DATA_BLOCK "Telegramindeling"
TITLE =
VERSION : 0.1


  STRUCT
   Telegram3 : STRUCT
    hoogwater : BOOL ;
    laagwater : BOOL ;
    water_op_vloer : BOOL ;
    lenspomp_1_stor : BOOL ;
    gereserveerd : BOOL ;
    niveaumeter_1_stor : BOOL ;
    analoge_ingang_1_stor : BOOL ;
    niveaumeter_2_stor : BOOL ;
    analoge_ingang_2_stor : BOOL ;
    verzamelstor_pompen : BOOL ;
    regenpompen_in : BOOL ;
    regenpompen_uit : BOOL ;
    inbraakalarm : BOOL ;
    debietmeter_stor : BOOL ;
    droogloop_elektrode : BOOL ;
    drukknop_herstel_stor : BOOL ;
   END_STRUCT ;
   Telegram4 : STRUCT
    pomp_1_thermistor_stor : BOOL ;
    pomp_1_terugmelding : BOOL ;
    pomp_1_looptijd_te_lang : BOOL ;
    pomp_1_thermische_stor : BOOL ;
    pomp_2_thermistor_stor : BOOL ;
    pomp_2_terugmelding : BOOL ;
    pomp_2_looptijd_te_lang : BOOL ;
    pomp_2_thermische_stor : BOOL ;
    pomp_3_thermistor_stor : BOOL ;
    pomp_3_terugmelding : BOOL ;
    pomp_3_looptijd_te_lang : BOOL ;
    pomp_3_thermische_stor : BOOL ;
    overstorthoogte_bereikt : BOOL ;
    gereserveerd1 : BOOL ;
    vlotterbal_kelder1_hoog : BOOL ;
    gereserveerd2 : BOOL ;
   END_STRUCT ;
   Telegram5 : STRUCT
    pomp_4_thermistor_stor : BOOL ;
    pomp_4_terugmelding : BOOL ;
    pomp_4_looptijd_te_lang : BOOL ;
    pomp_4_thermische_stor : BOOL ;
    pomp_5_thermistor_stor : BOOL ;
    pomp_5_terugmelding : BOOL ;
    pomp_5_looptijd_te_lang : BOOL ;
    pomp_5_thermische_stor : BOOL ;
    pomp_6_thermistor_stor : BOOL ;
    pomp_6_terugmelding : BOOL ;
    pomp_6_looptijd_te_lang : BOOL ;
    pomp_6_thermische_stor : BOOL ;
    procesafsluiter_stor : BOOL ;
    netwachter_stor : BOOL ;
    stuurstroom_stor : BOOL ;
    gereserveerd1 : BOOL ;
   END_STRUCT ;
   Telegram6 : STRUCT
    gereserveerd1 : BOOL ;
    gereserveerd2 : BOOL ;
    gereserveerd3 : BOOL ;
    gereserveerd4 : BOOL ;
    gereserveerd5 : BOOL ;
    gereserveerd6 : BOOL ;
    gereserveerd7 : BOOL ;
    gereserveerd8 : BOOL ;
    gereserveerd9 : BOOL ;
    gereserveerd10 : BOOL ;
    gereserveerd11 : BOOL ;
    gereserveerd12 : BOOL ;
    gereserveerd13 : BOOL ;
    gereserveerd14 : BOOL ;
    gereserveerd15 : BOOL ;
    gereserveerd16 : BOOL ;
   END_STRUCT ;
   Telegram7 : STRUCT
    gereserveerd1 : BOOL ;
    gereserveerd2 : BOOL ;
    gereserveerd3 : BOOL ;
    gereserveerd4 : BOOL ;
    gereserveerd5 : BOOL ;
    gereserveerd6 : BOOL ;
    gereserveerd7 : BOOL ;
    gereserveerd8 : BOOL ;
    gereserveerd9 : BOOL ;
    gereserveerd10 : BOOL ;
    gereserveerd11 : BOOL ;
    gereserveerd12 : BOOL ;
    gereserveerd13 : BOOL ;
    gereserveerd14 : BOOL ;
    gereserveerd15 : BOOL ;
    gereserveerd16 : BOOL ;
   END_STRUCT ;
   Telegram8 : STRUCT
    pomp_1_inbedrijf : BOOL ;
    pomp_2_inbedrijf : BOOL ;
    pomp_3_inbedrijf : BOOL ;
    pomp_4_inbedrijf : BOOL ;
    pomp_5_inbedrijf : BOOL ;
    pomp_6_inbedrijf : BOOL ;
    bedienpers_aanwezig : BOOL ;
    lenspomp_1_inbedrijf : BOOL ;
    regenmeter_puls : BOOL ;
    gereserveerd1 : BOOL ;
    gereserveerd2 : BOOL ;
    gereserveerd3 : BOOL ;
    gereserveerd4 : BOOL ;
    gereserveerd5 : BOOL ;
    gereserveerd6 : BOOL ;
    gereserveerd7 : BOOL ;
   END_STRUCT ;
   Telegram9 : STRUCT
    gereserveerd1 : BOOL ;
    gereserveerd2 : BOOL ;
    gereserveerd3 : BOOL ;
    gereserveerd4 : BOOL ;
    gereserveerd5 : BOOL ;
    gereserveerd6 : BOOL ;
    gereserveerd7 : BOOL ;
    gereserveerd8 : BOOL ;
    gereserveerd9 : BOOL ;
    gereserveerd10 : BOOL ;
    gereserveerd11 : BOOL ;
    gereserveerd12 : BOOL ;
    gereserveerd13 : BOOL ;
    gereserveerd14 : BOOL ;
    gereserveerd15 : BOOL ;
    gereserveerd16 : BOOL ;
   END_STRUCT ;
   Telegram10 : STRUCT
    gereserveerd : BOOL ;
    batterijspanning_laag : BOOL ;
    overstort_herstel : BOOL ;
    gereserveerd1 : BOOL ;
    gereserveerd2 : BOOL ;
    gereserveerd3 : BOOL ;
    gereserveerd4 : BOOL ;
    gereserveerd5 : BOOL ;
    gereserveerd6 : BOOL ;
    gereserveerd7 : BOOL ;
    gereserveerd8 : BOOL ;
    gereserveerd9 : BOOL ;
    gereserveerd10 : BOOL ;
    gereserveerd11 : BOOL ;
    gereserveerd12 : BOOL ;
    gereserveerd13 : BOOL ;
   END_STRUCT ;
   Telegram11 : STRUCT
    besturing_remote : BOOL ;
    besturing_lokaal : BOOL ;
    niveaumeter_1_actief : BOOL ;
    niveaumeter_2_actief : BOOL ;
    pomp_1_Auto : BOOL ;
    pomp_1_Hand : BOOL ;
    pomp_1_werksch_in : BOOL ;
    pomp_1_voorkeuze : BOOL ;
    pomp_2_Auto : BOOL ;
    pomp_2_Hand : BOOL ;
    pomp_2_werksch_in : BOOL ;
    pomp_2_voorkeuze : BOOL ;
    pomp_3_Auto : BOOL ;
    pomp_3_Hand : BOOL ;
    pomp_3_werksch_in : BOOL ;
    pomp_3_voorkeuze : BOOL ;
   END_STRUCT ;
   Telegram12 : STRUCT
    pomp_4_Auto : BOOL ;
    pomp_4_Hand : BOOL ;
    pomp_4_werksch_in : BOOL ;
    pomp_4_voorkeuze : BOOL ;
    pomp_5_Auto : BOOL ;
    pomp_5_Hand : BOOL ;
    pomp_5_werksch_in : BOOL ;
    pomp_5_voorkeuze : BOOL ;
    pomp_6_Auto : BOOL ;
    pomp_6_Hand : BOOL ;
    pomp_6_werksch_in : BOOL ;
    pomp_6_voorkeuze : BOOL ;
    reserve : BOOL ;
    lenspomp_1_Auto : BOOL ;
    lenspomp_1_Hand : BOOL ;
    lenspomp_1_werksch_in : BOOL ;
   END_STRUCT ;
   Telegram13 : STRUCT
    gereserveerd1 : BOOL ;
    gereserveerd2 : BOOL ;
    gereserveerd3 : BOOL ;
    gereserveerd4 : BOOL ;
    gereserveerd5 : BOOL ;
    gereserveerd6 : BOOL ;
    gereserveerd7 : BOOL ;
    gereserveerd8 : BOOL ;
    gereserveerd9 : BOOL ;
    gereserveerd10 : BOOL ;
    gereserveerd11 : BOOL ;
    gereserveerd12 : BOOL ;
    gereserveerd13 : BOOL ;
    gereserveerd14 : BOOL ;
    gereserveerd15 : BOOL ;
    gereserveerd16 : BOOL ;
   END_STRUCT ;
   Telegram14 : STRUCT
    Spanning_220_VAC : BOOL ;
    Spanning_24_VDC : BOOL ;
    gereserveerd1 : BOOL ;
    gereserveerd2 : BOOL ;
    gereserveerd3 : BOOL ;
    gereserveerd4 : BOOL ;
    gereserveerd5 : BOOL ;
    gereserveerd6 : BOOL ;
    gereserveerd7 : BOOL ;
    gereserveerd8 : BOOL ;
    gereserveerd9 : BOOL ;
    gereserveerd10 : BOOL ;
    gereserveerd11 : BOOL ;
    gereserveerd12 : BOOL ;
    gereserveerd13 : BOOL ;
    gereserveerd14 : BOOL ;
   END_STRUCT ;
Telegram21  :  STRUCT
niveaumeting_1  : WORD ;
niveaumeting_2  : WORD ;
regenmeter_niveau  : WORD ;
gereserveerd1  : WORD ;
gereserveerd2  : WORD ;
gereserveerd3  : WORD ;
gereserveerd4  : WORD ;
gereserveerd5  : WORD ;
END_STRUCT;
Telegram22  :  STRUCT
gereserveerd1  : WORD ;
gereserveerd2  : WORD ;
gereserveerd3  : WORD ;
gereserveerd4  : WORD ;
gereserveerd5  : WORD ;
gereserveerd6  : WORD ;
gereserveerd7  : WORD ;
gereserveerd8  : WORD ;
END_STRUCT;
Telegram23  :  STRUCT
debiet  : WORD ;
gereserveerd  : WORD ;
pomp_1_pompstroom  : WORD ;
pomp_2_pompstroom  : WORD ;
pomp_3_pompstroom  : WORD ;
pomp_4_pompstroom  : WORD ;
pomp_5_pompstroom  : WORD ;
pomp_6_pompstroom  : WORD ;
END_STRUCT;
Telegram24  :  STRUCT
gereserveerd1  : WORD ;
gereserveerd2  : WORD ;
gereserveerd3  : WORD ;
gereserveerd4  : WORD ;
gereserveerd5  : WORD ;
gereserveerd6  : WORD ;
gereserveerd7  : WORD ;
gereserveerd8  : WORD ;
END_STRUCT;
Telegram25  :  STRUCT
gereserveerd1  : WORD ;
gereserveerd2  : WORD ;
gereserveerd3  : WORD ;
gereserveerd4  : WORD ;
gereserveerd5  : WORD ;
gereserveerd6  : WORD ;
gereserveerd7  : WORD ;
gereserveerd8  : WORD ;
END_STRUCT;
Telegram31  :  STRUCT
pomp_1_bedrijfsuren  : WORD ;
pomp_2_bedrijfsuren  : WORD ;
pomp_3_bedrijfsuren  : WORD ;
pomp_4_bedrijfsuren  : WORD ;
pomp_5_bedrijfsuren  : WORD ;
pomp_6_bedrijfsuren  : WORD ;
kWh_totaal  : WORD ;
debiet_totaal  : WORD ;
END_STRUCT;
Telegram32  :  STRUCT
gereserveerd1  : WORD ;
gereserveerd2  : WORD ;
gereserveerd3  : WORD ;
gereserveerd4  : WORD ;
gereserveerd5  : WORD ;
regenmeter  : WORD ;
gereserveerd7  : WORD ;
gereserveerd8  : WORD ;
END_STRUCT;
Telegram33  :  STRUCT
gereserveerd1  : WORD ;
gereserveerd2  : WORD ;
gereserveerd3  : WORD ;
gereserveerd4  : WORD ;
gereserveerd5  : WORD ;
gereserveerd6  : WORD ;
gereserveerd7  : WORD ;
gereserveerd8  : WORD ;
END_STRUCT;

  END_STRUCT ;
BEGIN
   Telegram3.hoogwater := FALSE;
   Telegram3.laagwater := FALSE;
   Telegram3.water_op_vloer := FALSE;
   Telegram3.lenspomp_1_stor := FALSE;
   Telegram3.gereserveerd := FALSE;
   Telegram3.niveaumeter_1_stor := FALSE;
   Telegram3.analoge_ingang_1_stor := FALSE;
   Telegram3.niveaumeter_2_stor := FALSE;
   Telegram3.analoge_ingang_2_stor := FALSE;
   Telegram3.verzamelstor_pompen := FALSE;
   Telegram3.regenpompen_in := FALSE;
   Telegram3.regenpompen_uit := FALSE;
   Telegram3.inbraakalarm := FALSE;
   Telegram3.debietmeter_stor := FALSE;
   Telegram3.droogloop_elektrode := FALSE;
   Telegram3.drukknop_herstel_stor := FALSE;
   Telegram4.pomp_1_thermistor_stor := FALSE;
   Telegram4.pomp_1_terugmelding := FALSE;
   Telegram4.pomp_1_looptijd_te_lang := FALSE;
   Telegram4.pomp_1_thermische_stor := FALSE;
   Telegram4.pomp_2_thermistor_stor := FALSE;
   Telegram4.pomp_2_terugmelding := FALSE;
   Telegram4.pomp_2_looptijd_te_lang := FALSE;
   Telegram4.pomp_2_thermische_stor := FALSE;
   Telegram4.pomp_3_thermistor_stor := FALSE;
   Telegram4.pomp_3_terugmelding := FALSE;
   Telegram4.pomp_3_looptijd_te_lang := FALSE;
   Telegram4.pomp_3_thermische_stor := FALSE;
   Telegram4.overstorthoogte_bereikt := FALSE;
   Telegram4.gereserveerd1 := FALSE;
   Telegram4.vlotterbal_kelder1_hoog := FALSE;
   Telegram4.gereserveerd2 := FALSE;
   Telegram5.pomp_4_thermistor_stor := FALSE;
   Telegram5.pomp_4_terugmelding := FALSE;
   Telegram5.pomp_4_looptijd_te_lang := FALSE;
   Telegram5.pomp_4_thermische_stor := FALSE;
   Telegram5.pomp_5_thermistor_stor := FALSE;
   Telegram5.pomp_5_terugmelding := FALSE;
   Telegram5.pomp_5_looptijd_te_lang := FALSE;
   Telegram5.pomp_5_thermische_stor := FALSE;
   Telegram5.pomp_6_thermistor_stor := FALSE;
   Telegram5.pomp_6_terugmelding := FALSE;
   Telegram5.pomp_6_looptijd_te_lang := FALSE;
   Telegram5.pomp_6_thermische_stor := FALSE;
   Telegram5.procesafsluiter_stor := FALSE;
   Telegram5.netwachter_stor := FALSE;
   Telegram5.stuurstroom_stor := FALSE;
   Telegram5.gereserveerd1 := FALSE;
   Telegram6.gereserveerd1 := FALSE;
   Telegram6.gereserveerd2 := FALSE;
   Telegram6.gereserveerd3 := FALSE;
   Telegram6.gereserveerd4 := FALSE;
   Telegram6.gereserveerd5 := FALSE;
   Telegram6.gereserveerd6 := FALSE;
   Telegram6.gereserveerd7 := FALSE;
   Telegram6.gereserveerd8 := FALSE;
   Telegram6.gereserveerd9 := FALSE;
   Telegram6.gereserveerd10 := FALSE;
   Telegram6.gereserveerd11 := FALSE;
   Telegram6.gereserveerd12 := FALSE;
   Telegram6.gereserveerd13 := FALSE;
   Telegram6.gereserveerd14 := FALSE;
   Telegram6.gereserveerd15 := FALSE;
   Telegram6.gereserveerd16 := FALSE;
   Telegram7.gereserveerd1 := FALSE;
   Telegram7.gereserveerd2 := FALSE;
   Telegram7.gereserveerd3 := FALSE;
   Telegram7.gereserveerd4 := FALSE;
   Telegram7.gereserveerd5 := FALSE;
   Telegram7.gereserveerd6 := FALSE;
   Telegram7.gereserveerd7 := FALSE;
   Telegram7.gereserveerd8 := FALSE;
   Telegram7.gereserveerd9 := FALSE;
   Telegram7.gereserveerd10 := FALSE;
   Telegram7.gereserveerd11 := FALSE;
   Telegram7.gereserveerd12 := FALSE;
   Telegram7.gereserveerd13 := FALSE;
   Telegram7.gereserveerd14 := FALSE;
   Telegram7.gereserveerd15 := FALSE;
   Telegram7.gereserveerd16 := FALSE;
   Telegram8.pomp_1_inbedrijf := FALSE;
   Telegram8.pomp_2_inbedrijf := FALSE;
   Telegram8.pomp_3_inbedrijf := FALSE;
   Telegram8.pomp_4_inbedrijf := FALSE;
   Telegram8.pomp_5_inbedrijf := FALSE;
   Telegram8.pomp_6_inbedrijf := FALSE;
   Telegram8.bedienpers_aanwezig := FALSE;
   Telegram8.lenspomp_1_inbedrijf := FALSE;
   Telegram8.regenmeter_puls := FALSE;
   Telegram8.gereserveerd1 := FALSE;
   Telegram8.gereserveerd2 := FALSE;
   Telegram8.gereserveerd3 := FALSE;
   Telegram8.gereserveerd4 := FALSE;
   Telegram8.gereserveerd5 := FALSE;
   Telegram8.gereserveerd6 := FALSE;
   Telegram8.gereserveerd7 := FALSE;
   Telegram9.gereserveerd1 := FALSE;
   Telegram9.gereserveerd2 := FALSE;
   Telegram9.gereserveerd3 := FALSE;
   Telegram9.gereserveerd4 := FALSE;
   Telegram9.gereserveerd5 := FALSE;
   Telegram9.gereserveerd6 := FALSE;
   Telegram9.gereserveerd7 := FALSE;
   Telegram9.gereserveerd8 := FALSE;
   Telegram9.gereserveerd9 := FALSE;
   Telegram9.gereserveerd10 := FALSE;
   Telegram9.gereserveerd11 := FALSE;
   Telegram9.gereserveerd12 := FALSE;
   Telegram9.gereserveerd13 := FALSE;
   Telegram9.gereserveerd14 := FALSE;
   Telegram9.gereserveerd15 := FALSE;
   Telegram9.gereserveerd16 := FALSE;
   Telegram10.gereserveerd := FALSE;
   Telegram10.batterijspanning_laag := FALSE;
   Telegram10.overstort_herstel := FALSE;
   Telegram10.gereserveerd1 := FALSE;
   Telegram10.gereserveerd2 := FALSE;
   Telegram10.gereserveerd3 := FALSE;
   Telegram10.gereserveerd4 := FALSE;
   Telegram10.gereserveerd5 := FALSE;
   Telegram10.gereserveerd6 := FALSE;
   Telegram10.gereserveerd7 := FALSE;
   Telegram10.gereserveerd8 := FALSE;
   Telegram10.gereserveerd9 := FALSE;
   Telegram10.gereserveerd10 := FALSE;
   Telegram10.gereserveerd11 := FALSE;
   Telegram10.gereserveerd12 := FALSE;
   Telegram10.gereserveerd13 := FALSE;
   Telegram11.besturing_remote := FALSE;
   Telegram11.besturing_lokaal := FALSE;
   Telegram11.niveaumeter_1_actief := FALSE;
   Telegram11.niveaumeter_2_actief := FALSE;
   Telegram11.pomp_1_Auto := FALSE;
   Telegram11.pomp_1_Hand := FALSE;
   Telegram11.pomp_1_werksch_in := FALSE;
   Telegram11.pomp_1_voorkeuze := FALSE;
   Telegram11.pomp_2_Auto := FALSE;
   Telegram11.pomp_2_Hand := FALSE;
   Telegram11.pomp_2_werksch_in := FALSE;
   Telegram11.pomp_2_voorkeuze := FALSE;
   Telegram11.pomp_3_Auto := FALSE;
   Telegram11.pomp_3_Hand := FALSE;
   Telegram11.pomp_3_werksch_in := FALSE;
   Telegram11.pomp_3_voorkeuze := FALSE;
   Telegram12.pomp_4_Auto := FALSE;
   Telegram12.pomp_4_Hand := FALSE;
   Telegram12.pomp_4_werksch_in := FALSE;
   Telegram12.pomp_4_voorkeuze := FALSE;
   Telegram12.pomp_5_Auto := FALSE;
   Telegram12.pomp_5_Hand := FALSE;
   Telegram12.pomp_5_werksch_in := FALSE;
   Telegram12.pomp_5_voorkeuze := FALSE;
   Telegram12.pomp_6_Auto := FALSE;
   Telegram12.pomp_6_Hand := FALSE;
   Telegram12.pomp_6_werksch_in := FALSE;
   Telegram12.pomp_6_voorkeuze := FALSE;
   Telegram12.reserve := FALSE;
   Telegram12.lenspomp_1_Auto := FALSE;
   Telegram12.lenspomp_1_Hand := FALSE;
   Telegram12.lenspomp_1_werksch_in := FALSE;
   Telegram13.gereserveerd1 := FALSE;
   Telegram13.gereserveerd2 := FALSE;
   Telegram13.gereserveerd3 := FALSE;
   Telegram13.gereserveerd4 := FALSE;
   Telegram13.gereserveerd5 := FALSE;
   Telegram13.gereserveerd6 := FALSE;
   Telegram13.gereserveerd7 := FALSE;
   Telegram13.gereserveerd8 := FALSE;
   Telegram13.gereserveerd9 := FALSE;
   Telegram13.gereserveerd10 := FALSE;
   Telegram13.gereserveerd11 := FALSE;
   Telegram13.gereserveerd12 := FALSE;
   Telegram13.gereserveerd13 := FALSE;
   Telegram13.gereserveerd14 := FALSE;
   Telegram13.gereserveerd15 := FALSE;
   Telegram13.gereserveerd16 := FALSE;
   Telegram14.Spanning_220_VAC := FALSE;
   Telegram14.Spanning_24_VDC := FALSE;
   Telegram14.gereserveerd1 := FALSE;
   Telegram14.gereserveerd2 := FALSE;
   Telegram14.gereserveerd3 := FALSE;
   Telegram14.gereserveerd4 := FALSE;
   Telegram14.gereserveerd5 := FALSE;
   Telegram14.gereserveerd6 := FALSE;
   Telegram14.gereserveerd7 := FALSE;
   Telegram14.gereserveerd8 := FALSE;
   Telegram14.gereserveerd9 := FALSE;
   Telegram14.gereserveerd10 := FALSE;
   Telegram14.gereserveerd11 := FALSE;
   Telegram14.gereserveerd12 := FALSE;
   Telegram14.gereserveerd13 := FALSE;
   Telegram14.gereserveerd14 := FALSE;
   Telegram21.niveaumeting_1 := W#16#0;
Telegram21.niveaumeting_2 := W#16#0;
Telegram21.regenmeter_niveau := W#16#0;
Telegram21.gereserveerd1 := W#16#0;
Telegram21.gereserveerd2 := W#16#0;
Telegram21.gereserveerd3 := W#16#0;
Telegram21.gereserveerd4 := W#16#0;
Telegram21.gereserveerd5 := W#16#0;


Telegram22.gereserveerd1 := W#16#0;
Telegram22.gereserveerd2 := W#16#0;
Telegram22.gereserveerd3 := W#16#0;
Telegram22.gereserveerd4 := W#16#0;
Telegram22.gereserveerd5 := W#16#0;
Telegram22.gereserveerd6 := W#16#0;
Telegram22.gereserveerd7 := W#16#0;
Telegram22.gereserveerd8 := W#16#0;


Telegram23.debiet := W#16#0;
Telegram23.gereserveerd := W#16#0;
Telegram23.pomp_1_pompstroom := W#16#0;
Telegram23.pomp_2_pompstroom := W#16#0;
Telegram23.pomp_3_pompstroom := W#16#0;
Telegram23.pomp_4_pompstroom := W#16#0;
Telegram23.pomp_5_pompstroom := W#16#0;
Telegram23.pomp_6_pompstroom := W#16#0;


Telegram24.gereserveerd1 := W#16#0;
Telegram24.gereserveerd2 := W#16#0;
Telegram24.gereserveerd3 := W#16#0;
Telegram24.gereserveerd4 := W#16#0;
Telegram24.gereserveerd5 := W#16#0;
Telegram24.gereserveerd6 := W#16#0;
Telegram24.gereserveerd7 := W#16#0;
Telegram24.gereserveerd8 := W#16#0;


Telegram25.gereserveerd1 := W#16#0;
Telegram25.gereserveerd2 := W#16#0;
Telegram25.gereserveerd3 := W#16#0;
Telegram25.gereserveerd4 := W#16#0;
Telegram25.gereserveerd5 := W#16#0;
Telegram25.gereserveerd6 := W#16#0;
Telegram25.gereserveerd7 := W#16#0;
Telegram25.gereserveerd8 := W#16#0;


Telegram31.pomp_1_bedrijfsuren := W#16#0;
Telegram31.pomp_2_bedrijfsuren := W#16#0;
Telegram31.pomp_3_bedrijfsuren := W#16#0;
Telegram31.pomp_4_bedrijfsuren := W#16#0;
Telegram31.pomp_5_bedrijfsuren := W#16#0;
Telegram31.pomp_6_bedrijfsuren := W#16#0;
Telegram31.kWh_totaal := W#16#0;
Telegram31.debiet_totaal := W#16#0;


Telegram32.gereserveerd1 := W#16#0;
Telegram32.gereserveerd2 := W#16#0;
Telegram32.gereserveerd3 := W#16#0;
Telegram32.gereserveerd4 := W#16#0;
Telegram32.gereserveerd5 := W#16#0;
Telegram32.regenmeter := W#16#0;
Telegram32.gereserveerd7 := W#16#0;
Telegram32.gereserveerd8 := W#16#0;


Telegram33.gereserveerd1 := W#16#0;
Telegram33.gereserveerd2 := W#16#0;
Telegram33.gereserveerd3 := W#16#0;
Telegram33.gereserveerd4 := W#16#0;
Telegram33.gereserveerd5 := W#16#0;
Telegram33.gereserveerd6 := W#16#0;
Telegram33.gereserveerd7 := W#16#0;
Telegram33.gereserveerd8 := W#16#0;



END_DATA_BLOCK

